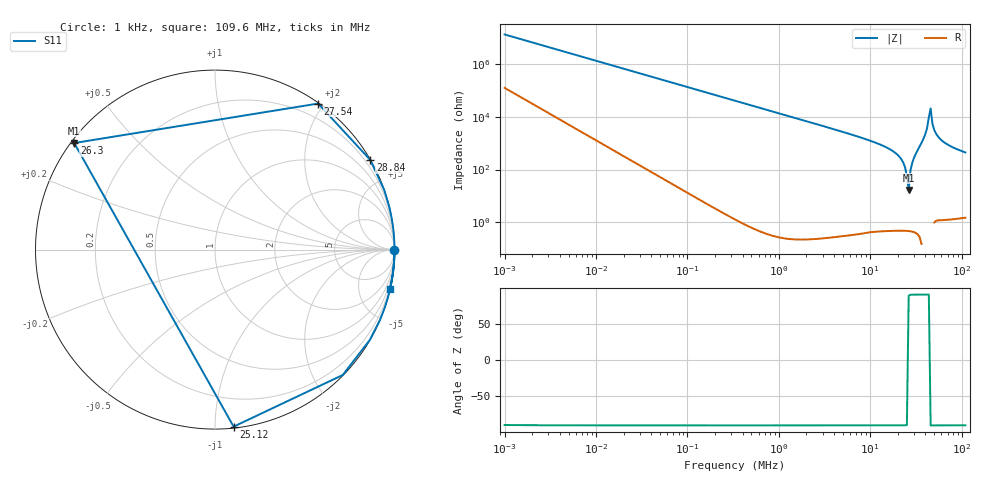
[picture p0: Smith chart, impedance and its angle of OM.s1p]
! EM Consulting and Software
! Touchstone file was created on 2026-03-09  16:25:52
# HZ S RI R 50.0000
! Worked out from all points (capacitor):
!   253 points, 1 kHz to 109.6 MHz, reference 50 ohm
!   read as one part to ground: C = 11.5 pF near 1.047 kHz
!   lowest |Z| = 16.8 ohm at 26.3 MHz (marker M1)
!   series resonance near 26.03 MHz, so ESL is about 3.3 uH
!   S11 on the Smith chart (normalised r, x): 1 kHz: open; 25.12 MHz: 0.01, -1.11; 26.3 MHz: 0.01, +0.34; 27.54 MHz: 0.01, +1.93; 28.84 MHz: 0.01, +3.73; 109.6 MHz: 0.03, -8.97
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1000  1 -7.2e-06
4365.158  1 -3.14e-05
18197.01  1 -0.000131
79432.82  1 -0.000572
331131.1  1 -0.00238
1445440  0.9999 -0.0104
6025596  0.999 -0.045
1.047129e7  0.9964 -0.0848
1.513561e7  0.9893 -0.145
1.737801e7  0.9816 -0.19
1.905461e7  0.9709 -0.2385
1.995262e7  0.9614 -0.2738
2.089296e7  0.9462 -0.3219
2.187762e7  0.9192 -0.392
2.290868e7  0.8628 -0.503
2.398833e7  0.7119 -0.6985
2.511886e7  0.1037 -0.9863
2.630268e7  -0.7845 0.5937
2.754229e7  0.5748 0.8137
2.884032e7  0.8648 0.4999
3.019952e7  0.9419 0.3344
3.162278e7  0.9711 0.238
3.311311e7  0.9845 0.1749
3.467369e7  0.9915 0.13
3.801894e7  0.9976 0.0689
4.365158e7  1 0.0104
5.011872e7  0.9995 -0.0314
1.096478e8  0.9747 -0.2201
